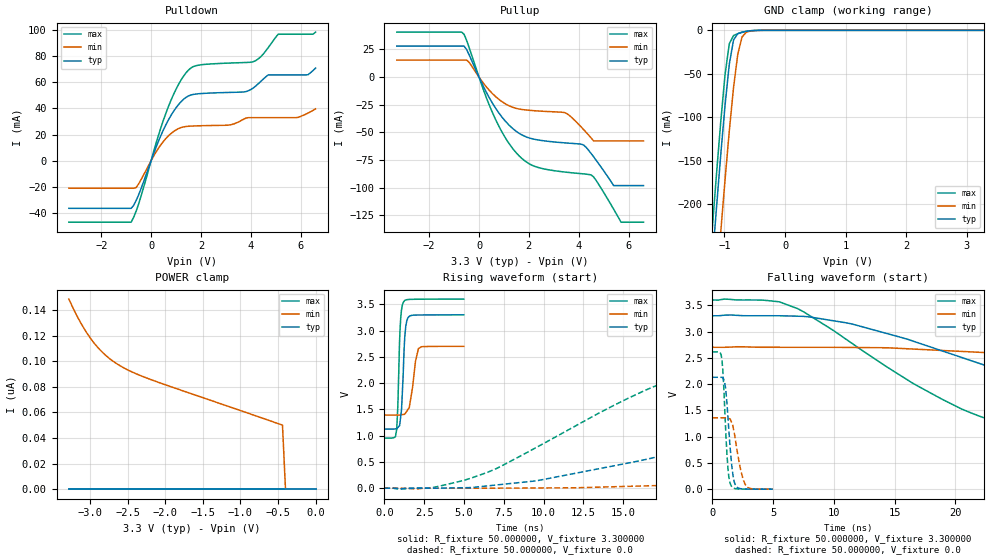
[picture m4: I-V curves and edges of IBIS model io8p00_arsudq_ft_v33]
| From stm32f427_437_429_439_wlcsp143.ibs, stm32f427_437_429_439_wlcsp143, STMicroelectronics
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|   Model io8p00_arsudq_ft_v33
[Model]  io8p00_arsudq_ft_v33
Model_type I/O
Polarity   Non-Inverting
Enable   Active-Low
Vinl =   0.990000V
Vinh =   2.310000V
Vmeas =  1.650000V
Cref =   50.000000pF
Rref =   100.000000M
Vref =   0.0V
C_comp   2.292100pF   2.219400pF   2.369900pF
[Temperature Range]   25.000000   0.125000k   -40.000000
[Pullup Reference]   3.300000V   2.700000V   3.600000V
[Pulldown Reference]   0.0V   0.0V   0.0V
[POWER Clamp Reference]   3.300000V   2.700000V   3.600000V
[GND Clamp Reference]   0.0V   0.0V   0.0V
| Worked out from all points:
|   slope of the pulldown table from 0 to 0.495 V, typ, clamps not added: 20.9 ohm
|   slope of the pullup table from 0 to 0.495 V, typ, clamps not added: 22.6 ohm
|   GND clamp passes 1 mA (typ) near -0.62 V on its own axis
|   rising waveform, R_fixture 50.000000, V_fixture 3.300000: 20-80 % time 191ps typ, 345ps min, 161ps max; typ from 1.12 V to 3.3 V
|   rising waveform, R_fixture 50.000000, V_fixture 0.0: 20-80 % time 19.7ns typ, 51.8ns min, 10.3ns max; typ from 0 V to 2.13 V
|   falling waveform, R_fixture 50.000000, V_fixture 3.300000: 20-80 % time 18.3ns typ, 38.8ns min, 11.3ns max; typ from 3.3 V to 1.12 V
|   falling waveform, R_fixture 50.000000, V_fixture 0.0: 20-80 % time 434ps typ, 652ps min, 341ps max; typ from 2.13 V to 0 V
[Pulldown]
|Voltage   I(typ)   I(min)   I(max)
-3.3V     -36.46mA   -21.09mA   -47.09mA
-800mV    -36.46mA   -21.09mA   -47.09mA
-600mV    -30.5mA    -20.54mA   -38.69mA
700mV     31.4mA     19.11mA    41.71mA
1.2V      45.15mA    25.37mA    61.75mA
1.6V      50.35mA    26.5mA     71.06mA
3.1V      52.28mA    27.26mA    74.76mA
4.1V      55.7mA     32.97mA    75.81mA
4.7V      65.71mA    32.97mA    86.64mA
5.1V      65.71mA    32.97mA    96.9mA
6.3V      65.88mA    36.51mA    96.9mA
6.6V      70.94mA    39.72mA    98.51mA
[Pullup]
|Voltage   I(typ)   I(min)   I(max)
-3.3V     28.03mA    15.43mA    40.69mA
-700mV    28.03mA    15.43mA    40.69mA
-400mV    20.31mA    13.47mA    26.93mA
600mV     -25.77mA   -16.23mA   -35.14mA
1.6V      -50.64mA   -28.81mA   -70.96mA
2.3V      -56.49mA   -30.48mA   -81.16mA
3.5V      -59.53mA   -32.65mA   -85.92mA
4.2V      -61.43mA   -47.47mA   -87.46mA
4.5V      -69.06mA   -55.01mA   -88.38mA
5.4V      -98mA      -57.7mA    -119.3mA
5.7V      -98mA      -57.7mA    -131.1mA
6.6V      -98mA      -57.7mA    -131.1mA
[GND_clamp]
|Voltage   I(typ)   I(min)   I(max)
-3.3V     -2.315A    -2.394A    -2.288A
-1.2V     -265.5mA   -356.1mA   -227.2mA
-1.13V    -202.6mA   -292.9mA   -164.1mA
-1.06V    -142.2mA   -231.2mA   -104.1mA
-990mV    -85.98mA   -171.6mA   -50.72mA
-920mV    -38.8mA    -115.5mA   -15.28mA
-850mV    -11.08mA   -65.6mA    -6.001mA
-780mV    -3.782mA   -27.42mA   -3.876mA
-710mV    -2.086mA   -7.69mA    -2.381mA
-640mV    -1.147mA   -2.118mA   -1.22mA
-570mV    -523.9uA   -798.4uA   -476.8uA
3.28V     0A         0A         0A
[POWER_clamp]
|Voltage   I(typ)   I(min)   I(max)
-3.28V    0A         148.5nA    0A
-3.2V     0A         138.6nA    0A
-3.12V    0A         129.7nA    0A
-3.04V    0A         122nA      0A
-2.96V    0A         115.3nA    0A
-2.8V     0A         105.1nA    0A
-2.6V     0A         96.44nA    0A
-2.4V     0A         90.52nA    0A
-2.16V    0A         84.97nA    0A
-440mV    0A         50.04nA    0A
-400mV    0A         0A         0A
0V        0A         0A         0A
[Ramp]
| variable   typ   min   max
dV/dt_r  1.27740/19.66065n   0.81588/51.85157n   1.56732/10.25437n
dV/dt_f  1.30602/18.31746n   0.78510/38.98223n   1.58792/11.32902n
R_load = 50.000000
[Rising Waveform]
R_fixture= 50.000000
V_fixture= 3.300000
V_fixture_min= 2.700000
V_fixture_max= 3.600000
|time   V(typ)   V(min)   V(max)
0s        1.124V     1.392V     953.5mV
770.8ps   1.133V     1.392V     1.12V
840.8ps   1.154V     1.391V     1.557V
981ps     1.257V     1.393V     3.022V
1.081ns   1.536V     1.398V     3.409V
1.201ns   2.36V      1.403V     3.545V
1.281ns   2.894V     1.41V      3.573V
1.401ns   3.183V     1.464V     3.588V
2.142ns   3.296V     2.659V     3.597V
4.985ns   3.3V       2.7V       3.6V
[Rising Waveform]
R_fixture= 50.000000
V_fixture= 0.0
V_fixture_min= 0.0
V_fixture_max= 0.0
|time   V(typ)   V(min)   V(max)
0s        120.5nV    244.5nV    640.3nV
3.003ns   -387.2uV   -326.2uV   9.196mV
6.507ns   43.76mV    -35.1uV    305.3mV
19.02ns   728.1mV    64.28mV    2.165V
30.53ns   1.502V     230.7mV    2.531V
39.54ns   1.886V     379.3mV    2.579V
54.05ns   2.052V     654mV      2.604V
86.59ns   2.116V     1.109V     2.612V
117.1ns   2.129V     1.299V     2.612V
249.2ns   2.129V     1.359V     2.612V
[Falling Waveform]
R_fixture= 50.000000
V_fixture= 3.300000
V_fixture_min= 2.700000
V_fixture_max= 3.600000
|time   V(typ)   V(min)   V(max)
0s        3.3V       2.7V       3.6V
4.505ns   3.3V       2.7V       3.59V
7.007ns   3.292V     2.7V       3.436V
16.52ns   2.818V     2.667V     2.013V
22.52ns   2.351V     2.598V     1.345V
32.03ns   1.674V     2.408V     1.066V
46.55ns   1.272V     2.066V     996.7mV
65.07ns   1.177V     1.695V     967.3mV
85.09ns   1.147V     1.532V     956.1mV
249.2ns   1.124V     1.392V     953.5mV
[Falling Waveform]
R_fixture= 50.000000
V_fixture= 0.0
V_fixture_min= 0.0
V_fixture_max= 0.0
|time   V(typ)   V(min)   V(max)
0s        2.129V     1.359V     2.612V
790.8ps   2.125V     1.358V     2.461V
1.001ns   2.046V     1.358V     1.623V
1.201ns   1.637V     1.357V     661.2mV
1.341ns   1.177V     1.346V     264.2mV
1.512ns   664mV      1.312V     85.63mV
1.882ns   87.3mV     963.8mV    10.08mV
2.272ns   11.18mV    427.3mV    2.461mV
2.693ns   2.855mV    92.74mV    1.223mV
4.985ns   120.5nV    244.5nV    640.3nV
